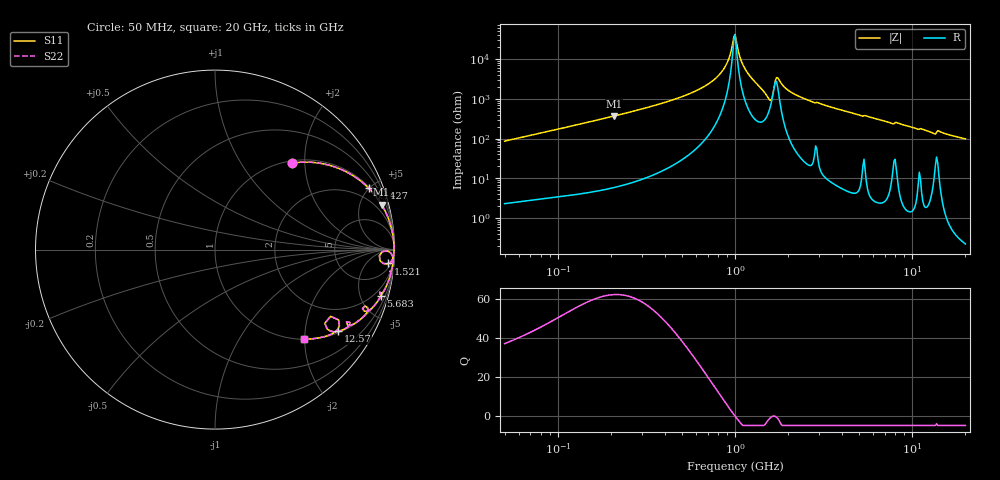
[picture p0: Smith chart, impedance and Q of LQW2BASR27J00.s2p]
!Murata Part Number: LQW2BASR27J00
!These Parameters are Measured in Series Mode Connection
!  o--[Z]--o
!Port1  Port2
!  o-------o
!Freq. Start=50[MHz] Stop=20[GHz], 401[Steps]
# Hz S RI R 50
!Freq.(Hz) S11(Real) S11(Imag) S21(Real) S21(Imag) S12(Real) S12(Imag) S22(Real) S22(Imag)
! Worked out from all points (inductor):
!   401 points, 50 MHz to 20 GHz, reference 50 ohm
!   read as one part in series: L = 274 nH near 51.52 MHz
!   highest Q = 62.4 at 207.5 MHz (marker M1), where L = 283 nH
!   self-resonance near 985.1 MHz
!   S11 on the Smith chart (normalised r, x): 50 MHz: 1.05, +1.73; 142.7 MHz: 1.09, +4.98; 1.521 GHz: 9, -22; 5.683 GHz: 1.09, -7.09; 12.57 GHz: 1.05, -2.99; 20 GHz: 1.00, -1.98
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5e7  0.4301 0.4818  0.5699 -0.4818  0.5699 -0.4818  0.4301 0.4818
1.364002e8  0.8451 0.3532  0.1549 -0.3532  0.1549 -0.3532  0.8451 0.3532
1.426693e8  0.8567 0.3419  0.1433 -0.3419  0.1433 -0.3419  0.8567 0.3419
2.074719e8  0.9283 0.2501  0.0717 -0.2501  0.0717 -0.2501  0.9283 0.2501
3.721004e8  0.9792 0.1333  0.0208 -0.1333  0.0208 -0.1333  0.9792 0.1333
5.831961e8  0.9933 0.0667  0.00668 -0.0667  0.00668 -0.0667  0.9933 0.0667
7.636728e8  0.9968 0.0326  0.00323 -0.0326  0.00323 -0.0326  0.9968 0.0326
8.870719e8  0.9976 0.0144  0.00244 -0.0144  0.00244 -0.0144  0.9976 0.0144
9.278425e8  0.9976 0.00887  0.00236 -0.00887  0.00236 -0.00887  0.9976 0.00887
9.70487e8  0.9977 0.00334  0.00235 -0.00334  0.00235 -0.00334  0.9977 0.00334
1e9  0.9976 -0.000393  0.00239 0.000393  0.00239 0.000393  0.9976 -0.000393
1.077769e9  0.9973 -0.00995  0.00269 0.00995  0.00269 0.00995  0.9973 -0.00995
1.144317e9  0.9968 -0.018  0.00318 0.018  0.00318 0.018  0.9968 -0.018
1.521052e9  0.9662 -0.0772  0.0338 0.0772  0.0338 0.0772  0.9662 -0.0772
1.590961e9  0.9188 -0.0606  0.0812 0.0606  0.0812 0.0606  0.9188 -0.0606
1.740566e9  0.9822 -0.023  0.0178 0.023  0.0178 0.023  0.9822 -0.023
2.05233e9  0.9919 -0.0657  0.00812 0.0657  0.00812 0.0657  0.9919 -0.0657
2.728004e9  0.9831 -0.1161  0.0169 0.1161  0.0169 0.1161  0.9831 -0.1161
5.683258e9  0.9237 -0.2596  0.0763 0.2596  0.0763 0.2596  0.9237 -0.2596
7.442007e9  0.8616 -0.3368  0.1384 0.3368  0.1384 0.3368  0.8616 -0.3368
1.257102e10  0.6872 -0.455  0.3128 0.455  0.3128 0.455  0.6872 -0.455
2e10  0.4941 -0.4988  0.5059 0.4988  0.5059 0.4988  0.4941 -0.4988
